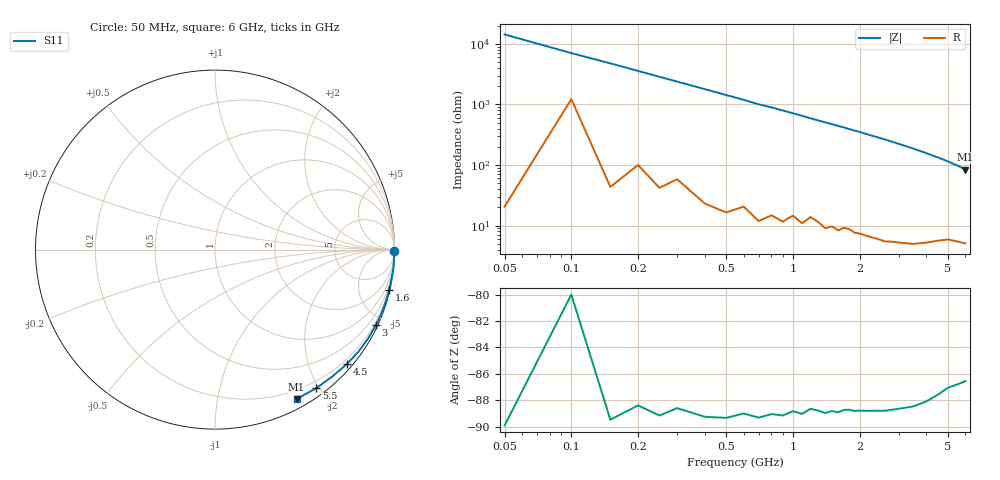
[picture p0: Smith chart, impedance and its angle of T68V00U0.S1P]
! SIEMENS Discrete & RF Semiconductors
! BAT62
! Si Schottky Diode in SOT143
! VR = 8 V
! S-Parameters:  February  1997
# GHz  S  MA  R  50
!  f  S11
! GHz  MAG  ANG
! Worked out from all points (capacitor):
!   34 points, 50 MHz to 6 GHz, reference 50 ohm
!   read as one part to ground: C = 222 fF near 50 MHz
!   lowest |Z| = 84.1 ohm at 6 GHz (marker M1)
!   S11 on the Smith chart (normalised r, x): 50 MHz: open; 1.6 GHz: 0.17, -8.84; 3 GHz: 0.10, -4.47; 4.5 GHz: 0.11, -2.67; 5.5 GHz: 0.11, -1.97; 6 GHz: 0.10, -1.68
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0.05  1 -0.4
0.1  0.9975 -0.8
0.15  0.9998 -1.2
0.2  0.9992 -1.6
0.4  0.9993 -3.2
0.6  0.9986 -4.8
0.7  0.9988 -5.7
0.8  0.9982 -6.4
0.9  0.9982 -7.2
1  0.9972 -8.0
1.1  0.9974 -8.8
1.2  0.9961 -9.7
1.4  0.9965 -11.3
1.6  0.9958 -12.9
1.7  0.9948 -13.7
1.8  0.9944 -14.6
2  0.9941 -16.2
2.2  0.9936 -18.0
2.4  0.993 -19.7
2.6  0.9924 -21.5
2.8  0.9912 -23.3
3  0.9901 -25.2
3.5  0.9867 -30.1
4  0.9809 -35.4
4.5  0.9728 -41.0
5  0.9631 -47.1
5.5  0.9562 -53.8
6  0.9486 -61.4
